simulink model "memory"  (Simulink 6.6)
settings: Solver=ode45  StartTime=0.0  StopTime=25.0  RelTol=1e-3
undefined symbols (not defined in the file or in its folder): Bit, Location, Lower, netlist, Width
libraries: xbsIndex_r4 x26, adlibrary2 x2

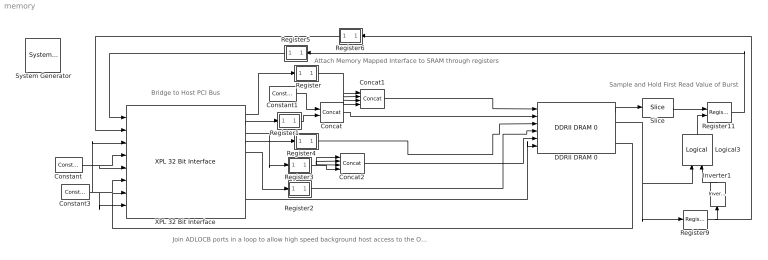
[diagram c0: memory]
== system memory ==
  note: Bridge to Host PCI Bus
  note: Attach Memory Mapped Interface to SRAM through registers
  note: Join ADLOCB ports in a loop to allow high speed background host access to the Off Chip Ram
  note: Sample and Hold First Read Value of Burst
  " System Generator" : xbsIndex_r4/ System Generator  Tag=genX  SystemSampleTime=-1  xilinxfamily=virtex5  part=xc5vsx95t  speed=-1  package=ff1136  synthesis_tool=XST  directory=./netlist  testbench=off  simulink_period=1  sysclk_period=6  incr_netlist=off  trim_vbits=Everywhere in SubSystem  dbl_ovrd=According to Block Masks  core_generation=According to Block Masks  run_coregen=off  deprecated_control=off  eval_field=0  block_type=sysgen
  Concat : xbsIndex_r4/Concat  num_inputs=2  dbl_ovrd=off  block_type=concat
  Concat1 : xbsIndex_r4/Concat  num_inputs=4  dbl_ovrd=off  block_type=concat
  Concat2 : xbsIndex_r4/Concat  num_inputs=4  dbl_ovrd=off  block_type=concat
  Constant : xbsIndex_r4/Constant  arith_type=Boolean  const=0  n_bits=1  bin_pt=0  explicit_period=on  period=1  equ=P=C  opselect=C  inp2=PCIN>>17  opr=+  inp1=P  carry=CIN  dbl_ovrd=off  block_type=constant
  Constant1 : xbsIndex_r4/Constant  arith_type=Unsigned  const=0  n_bits=12  bin_pt=0  explicit_period=on  period=1  equ=P=C  opselect=C  inp2=PCIN>>17  opr=+  inp1=P  carry=CIN  dbl_ovrd=off  block_type=constant
  Constant3 : xbsIndex_r4/Constant  arith_type=Unsigned  const=0  n_bits=32  bin_pt=0  explicit_period=on  period=1  equ=P=C  opselect=C  inp2=PCIN>>17  opr=+  inp1=P  carry=CIN  dbl_ovrd=off  block_type=constant
  DDRII DRAM 0 : adlibrary2/ADM-XRC-5T1/DDRII DRAM 0  SystemSampleTime=-1  rate=1
  Inverter1 : xbsIndex_r4/Inverter  Orientation=up  en=off  latency=0  dbl_ovrd=off  block_type=inv
  Logical3 : xbsIndex_r4/Logical  Orientation=up  logical_function=AND  inputs=2  en=off  latency=0  precision=Full  arith_type=Unsigned  n_bits=8  bin_pt=2  align_bp=on  dbl_ovrd=off  block_type=logical
  Register : Subsystem
  Register1 : Subsystem
  Register11 : xbsIndex_r4/Register  init=0  rst=off  en=on  dbl_ovrd=off  block_type=register
  Register2 : Subsystem
  Register3 : Subsystem
  Register4 : Subsystem
  Register5 : Subsystem  Orientation=left
  Register6 : Subsystem  Orientation=left
  Register9 : xbsIndex_r4/Register  init=0  rst=off  en=off  dbl_ovrd=off  block_type=register
  Slice : xbsIndex_r4/Slice  nbits=32  boolean_output=off  mode=Lower Bit Location + Width  bit1=0  base1=MSB of Input  bit0=0  base0=LSB of Input  dbl_ovrd=off  block_type=slice
  XPL 32 Bit Interface : adlibrary2/ADM-XPL/XPL 32 Bit Interface  SystemSampleTime=-1  program='slave_write 0x0 0x1234;slave_read 0x0'  clock_ratio=1.5  sstep_clk_sel_default=0
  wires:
  Constant/1 -> XPL 32 Bit Interface/5, XPL 32 Bit Interface/4
  Constant3/1 -> XPL 32 Bit Interface/3, XPL 32 Bit Interface/6, XPL 32 Bit Interface/8
  XPL 32 Bit Interface/5 -> Register2/1(in0)
  XPL 32 Bit Interface/2 -> Register1/1(in0)
  XPL 32 Bit Interface/1 -> Register/1(in0)
  Register/1(out0) -> Concat1/1, Concat1/2, Concat1/3, Concat1/4
  Register4/1(out0) -> DDRII DRAM 0/3
  Constant1/1 -> Concat/1
  Register1/1(out0) -> Concat/2
  Register5/1(out0) -> XPL 32 Bit Interface/1
  Register6/1(out0) -> XPL 32 Bit Interface/2
  Register3/1(out0) -> Concat2/1, Concat2/2, Concat2/3, Concat2/4
  XPL 32 Bit Interface/4 -> Register4/1(in0)
  XPL 32 Bit Interface/3 -> Register3/1(in0)
  DDRII DRAM 0/4 -> XPL 32 Bit Interface/7
  XPL 32 Bit Interface/10 -> DDRII DRAM 0/6
  Register2/1(out0) -> DDRII DRAM 0/4
  DDRII DRAM 0/1 -> Slice/1
  Slice/1 -> Register11/1
  Logical3/1 -> Register11/2
  Inverter1/1 -> Logical3/2
  DDRII DRAM 0/2 -> Register9/1, Logical3/1
  Register9/1 -> Inverter1/1, Register6/1(in0)
  Register11/1 -> Register5/1(in0)
  Concat2/1 -> DDRII DRAM 0/5
  Concat1/1 -> DDRII DRAM 0/1
  Concat/1 -> DDRII DRAM 0/2

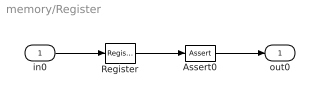
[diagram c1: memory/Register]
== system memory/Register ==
  in0 : Inport
  Assert0 : xbsIndex_r4/Assert  assert_type=off  type_source=Explicitly  arith_type="Signed  (2's comp)"  n_bits=16  bin_pt=14  assert_rate=on  rate_source=Explicitly  period=1  output_port=on  block_type=assert
  Register : xbsIndex_r4/Register  init=0  rst=off  en=off  dbl_ovrd=off  block_type=register
  out0 : Outport
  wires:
  in0/1 -> Register/1
  Register/1 -> Assert0/1
  Assert0/1 -> out0/1

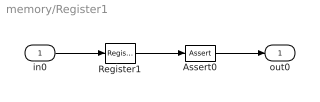
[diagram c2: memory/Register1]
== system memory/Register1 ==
  in0 : Inport
  Assert0 : xbsIndex_r4/Assert  assert_type=off  type_source=Explicitly  arith_type="Signed  (2's comp)"  n_bits=16  bin_pt=14  assert_rate=on  rate_source=Explicitly  period=1  output_port=on  block_type=assert
  Register1 : xbsIndex_r4/Register  init=0  rst=off  en=off  dbl_ovrd=off  block_type=register
  out0 : Outport
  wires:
  in0/1 -> Register1/1
  Register1/1 -> Assert0/1
  Assert0/1 -> out0/1

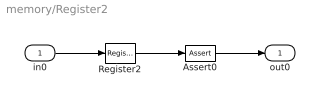
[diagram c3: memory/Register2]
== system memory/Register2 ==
  in0 : Inport
  Assert0 : xbsIndex_r4/Assert  assert_type=off  type_source=Explicitly  arith_type="Signed  (2's comp)"  n_bits=16  bin_pt=14  assert_rate=on  rate_source=Explicitly  period=1  output_port=on  block_type=assert
  Register2 : xbsIndex_r4/Register  init=0  rst=off  en=off  dbl_ovrd=off  block_type=register
  out0 : Outport
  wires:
  in0/1 -> Register2/1
  Register2/1 -> Assert0/1
  Assert0/1 -> out0/1

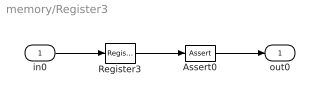
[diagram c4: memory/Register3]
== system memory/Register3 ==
  in0 : Inport
  Assert0 : xbsIndex_r4/Assert  assert_type=off  type_source=Explicitly  arith_type="Signed  (2's comp)"  n_bits=16  bin_pt=14  assert_rate=on  rate_source=Explicitly  period=1  output_port=on  block_type=assert
  Register3 : xbsIndex_r4/Register  init=0  rst=off  en=off  dbl_ovrd=off  block_type=register
  out0 : Outport
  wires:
  in0/1 -> Register3/1
  Register3/1 -> Assert0/1
  Assert0/1 -> out0/1

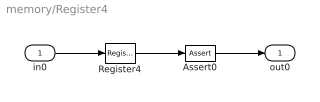
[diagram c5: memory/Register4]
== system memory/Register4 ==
  in0 : Inport
  Assert0 : xbsIndex_r4/Assert  assert_type=off  type_source=Explicitly  arith_type="Signed  (2's comp)"  n_bits=16  bin_pt=14  assert_rate=on  rate_source=Explicitly  period=1  output_port=on  block_type=assert
  Register4 : xbsIndex_r4/Register  init=0  rst=off  en=off  dbl_ovrd=off  block_type=register
  out0 : Outport
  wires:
  in0/1 -> Register4/1
  Register4/1 -> Assert0/1
  Assert0/1 -> out0/1

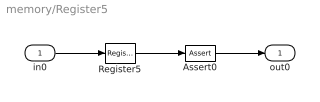
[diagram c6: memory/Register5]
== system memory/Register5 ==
  in0 : Inport
  Assert0 : xbsIndex_r4/Assert  assert_type=off  type_source=Explicitly  arith_type="Signed  (2's comp)"  n_bits=16  bin_pt=14  assert_rate=on  rate_source=Explicitly  period=1  output_port=on  block_type=assert
  Register5 : xbsIndex_r4/Register  init=0  rst=off  en=off  dbl_ovrd=off  block_type=register
  out0 : Outport
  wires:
  in0/1 -> Register5/1
  Register5/1 -> Assert0/1
  Assert0/1 -> out0/1

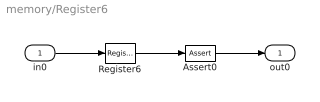
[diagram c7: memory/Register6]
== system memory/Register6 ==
  in0 : Inport
  Assert0 : xbsIndex_r4/Assert  assert_type=off  type_source=Explicitly  arith_type="Signed  (2's comp)"  n_bits=16  bin_pt=14  assert_rate=on  rate_source=Explicitly  period=1  output_port=on  block_type=assert
  Register6 : xbsIndex_r4/Register  init=0  rst=off  en=off  dbl_ovrd=off  block_type=register
  out0 : Outport
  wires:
  in0/1 -> Register6/1
  Register6/1 -> Assert0/1
  Assert0/1 -> out0/1
